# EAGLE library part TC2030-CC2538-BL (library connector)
Tag connect programmer for the CC2538 bootloader. The RX/TX switch happens on the programmer board, so when using this connect the TX pin to the TX pin on the CC2538 and same for the RX.
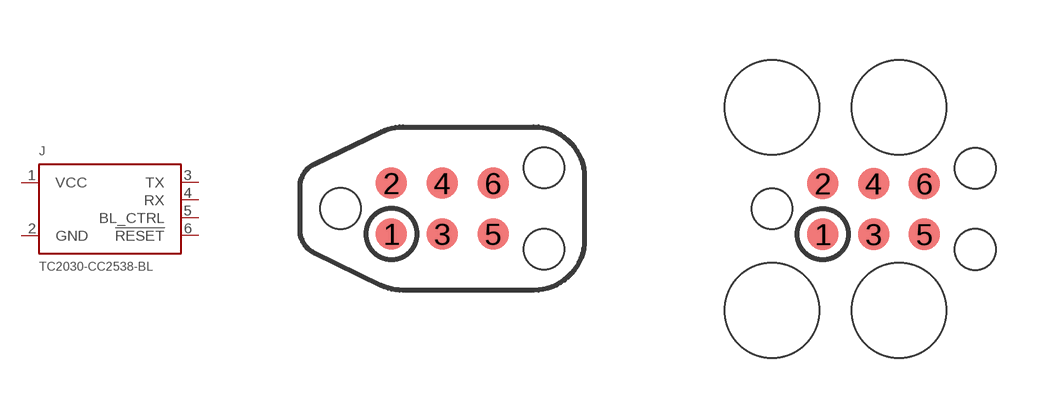
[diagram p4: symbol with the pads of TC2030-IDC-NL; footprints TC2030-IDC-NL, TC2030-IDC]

Designator prefix J

## TC2030-CC2538-BL-NL  [TC2030-IDC-NL]
1  VCC
2  GND
3  TX
4  RX
5  BL_CTRL
6  !RESET

## TC2030-CC2538-BL  [TC2030-IDC]
Pads as for TC2030-IDC-NL

## Footprint TC2030-IDC-NL (pad centres in mm)
The TC2030-IDC-NL is our "No Legs" 6-pin Plug-of-Nails Cable
smd 0.787 x 0.787: 1 -1.27,-0.635; 2 -1.27,0.635; 3 0,-0.635; 4 0,0.635; 5 1.27,-0.635; 6 1.27,0.635
hole 1.016 at -2.54,0
hole 1.016 at 2.54,1.016
hole 1.016 at 2.54,-1.016

## Footprint TC2030-IDC (pad centres in mm)
Tag Connect TC2030-IDC
smd 0.787 x 0.787: 1 -1.27,-0.635; 2 -1.27,0.635; 3 0,-0.635; 4 0,0.635; 5 1.27,-0.635; 6 1.27,0.635
hole 2.375 at -2.54,2.54
hole 2.375 at 0.635,2.54
hole 2.375 at 0.635,-2.54
hole 2.375 at -2.54,-2.54
hole 1.016 at -2.54,0
hole 1.016 at 2.54,1.016
hole 1.016 at 2.54,-1.016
